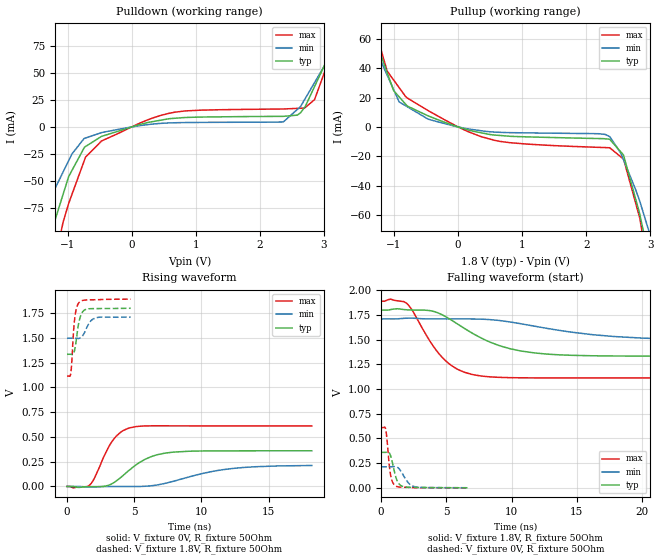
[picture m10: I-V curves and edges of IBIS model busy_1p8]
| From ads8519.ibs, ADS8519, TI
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|   busy_1p8 Model
[Model]   busy_1p8
Model_type   Output
Polarity   Non-Inverting
Vmeas = 0.9
Vref = 0.9
Cref = 5pF
Rref = 50
|   typ   min   max
|   (nom PVT)   (Fast PVT)   (slow PVT)
| C_comp by Frequency method (F=29Mhz)
|Average
C_comp   6.065e-12   5.169e-12   6.997e-12
|ON state : BUFFER OUTPUT TURNED HIGH
|C_comp   6.065e-12   5.169e-12   6.997e-12
|OFF state: BUFFER OUTPUT TURNED LOW
|C_comp   8.060e-12   7.497e-12   8.615e-12
| C_comp by LC Tank method (L=1nH)
| Resonant frequency (Hz)  2.8e9   3.07e9   2.58e9
|C_comp   3.227e-12   2.692e-12   3.80e-12
| Where nom  PVT is Nominal Process,  1.8V,  32C
|   Fast PVT is Strong Process,   1.89V,  -40C
|   Slow PVT is Weak Process,   1.71V,  92C
[Voltage Range]   1.8   1.71   1.89
|Ambient Temperature   25   85   -40
|Junction Temperature
[Temperature Range]   32   92   -40
[Pullup Reference]   1.8   1.71   1.89
[Pulldown Reference]   0   0   0
[Power Clamp Reference]   1.8   1.71   1.89
[GND Clamp Reference]   0   0   0
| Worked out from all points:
|   slope of the pulldown table from 0 to 0.27 V, typ, clamps not added: 62.8 ohm
|   slope of the pullup table from 0 to 0.27 V, typ, clamps not added: 83.6 ohm
|   falling waveform, V_fixture 1.8V, R_fixture 50Ohm: 20-80 % time 4.1ns typ, 6.77ns min, 2.44ns max; typ from 1.8 V to 1.33 V
|   rising waveform, V_fixture 0V, R_fixture 50Ohm: 20-80 % time 2.22ns typ, 3.97ns min, 1.37ns max; typ from 0 V to 0.36 V
|   rising waveform, V_fixture 1.8V, R_fixture 50Ohm: 20-80 % time 335ps typ, 500ps min, 252ps max; typ from 1.33 V to 1.8 V
|   falling waveform, V_fixture 0V, R_fixture 50Ohm: 20-80 % time 421ps typ, 632ps min, 289ps max; typ from 0.36 V to 0.001 V
[Pulldown]
|   Voltage   I(typ)   I(min)   I(max)
-1.8V     -215.3mA   -142.8mA   -308.6mA
-1.276V   -101mA     -66.35mA   -144.6mA
-1.07V    -62.1mA    -41.54mA   -87.79mA
-982.8mV  -45.72mA   -31.06mA   -70.51mA
-742.1mV  -19.31mA   -10.67mA   -31.46mA
-470.6mV  -8.722mA   -5.223mA   -12.94mA
574.6mV   7.501mA    3.675mA    12.46mA
2.365V    9.765mA    4.604mA    16.56mA
2.583V    10.91mA    16.15mA    17.13mA
2.852V    37.28mA    40.9mA     25.21mA
3.42V     109.2mA    98.28mA    117.8mA
3.6V      130mA      116.5mA    147.1mA
[Pullup]
|   Voltage   I(typ)   I(min)   I(max)
-1.8V     120.4mA    103mA      143.1mA
-1.71V    110.3mA    94.18mA    129.4mA
-1.108V   37.09mA    35.36mA    38.19mA
-1.006V   24.77mA    25.47mA    32mA
-920mV    20.5mA     17.05mA    26.8mA
-470.3mV  7.592mA    5.362mA    11.19mA
591.6mV   -5.604mA   -3.564mA   -9.333mA
2.362V    -8.392mA   -6.49mA    -14.18mA
2.582V    -19.48mA   -22.54mA   -21.96mA
2.839V    -60.61mA   -51.34mA   -63.11mA
3.081V    -109.6mA   -85.9mA    -131.1mA
3.6V      -223.7mA   -160.1mA   -294.7mA
[Ramp]
R_load = 50
|   typ   min   max
dV/dt_r   0.21588/2.20671e-09   0.128164/4.0361e-09   0.366666/1.37719e-09
dV/dt_f   0.279983/4.09846e-09   0.127933/6.70146e-09   0.466188/2.43882e-09
[Falling Waveform]
V_fixture = 1.8V
V_fixture_min = 1.71V
V_fixture_max = 1.89V
R_fixture = 50Ohm
|   Time   V(typ)   V(min)   V(max)
0s        1.8V       1.71V      1.89V
720ps     1.805V     1.71V      1.911V
1.92ns    1.803V     1.717V     1.872V
4.68ns    1.752V     1.71V      1.321V
5.8ns     1.663V     1.71V      1.205V
7.14ns    1.554V     1.71V      1.144V
9.38ns    1.427V     1.689V     1.117V
12.62ns   1.355V     1.617V     1.113V
19.96ns   1.334V     1.517V     1.113V
30ns      1.333V     1.497V     1.113V
[Rising Waveform]
V_fixture = 0V
V_fixture_min = 0V
V_fixture_max = 0V
R_fixture = 50Ohm
|   Time   V(typ)   V(min)   V(max)
0s        744.2pV    937.3pV    609.4pV
1.72ns    -1.763mV   -6.326mV   19.15mV
2.06ns    -1.867mV   -4.018mV   89.25mV
3.38ns    30.13mV    -721.6uV   459.4mV
4.02ns    92.96mV    -858.8uV   549.9mV
4.64ns    165.2mV    -889.2uV   590.2mV
6.22ns    298.4mV    6.348mV    611.5mV
7.9ns     346.4mV    51.66mV    611.4mV
12.32ns   359.5mV    181.5mV    611.1mV
18.22ns   359.8mV    211.6mV    611.1mV
[Rising Waveform]
V_fixture = 1.8V
V_fixture_min = 1.71V
V_fixture_max = 1.89V
R_fixture = 50Ohm
|   Time   V(typ)   V(min)   V(max)
0s        1.333V     1.495V     1.113V
280ps     1.333V     1.496V     1.141V
340ps     1.332V     1.496V     1.224V
500ps     1.344V     1.496V     1.59V
580ps     1.383V     1.495V     1.702V
720ps     1.509V     1.494V     1.805V
900ps     1.667V     1.494V     1.856V
1.28ns    1.778V     1.547V     1.879V
2.12ns    1.794V     1.7V       1.884V
4.74ns    1.798V     1.708V     1.89V
[Falling Waveform]
V_fixture = 0V
V_fixture_min = 0V
V_fixture_max = 0V
R_fixture = 50Ohm
|   Time   V(typ)   V(min)   V(max)
0s        359.8mV    213.6mV    611.1mV
340ps     359.6mV    213.5mV    595.5mV
420ps     360.8mV    213.4mV    522.5mV
700ps     333.8mV    213.5mV    146.6mV
860ps     256.3mV    214.5mV    62.48mV
1.06ns    139.1mV    215.3mV    24.32mV
1.5ns     24.34mV    171.7mV    7.75mV
2.02ns    7.199mV    60.3mV     4.971mV
2.5ns     4.844mV    14.21mV    3.035mV
6.62ns    739.9uV    1.537mV    86.39uV
